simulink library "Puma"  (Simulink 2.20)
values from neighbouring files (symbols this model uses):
  a = input('Inserisci il dato da graficare [1=PIDNL 2=PD 3=PID]: ')    [grp.m]    (also in grp1.m = input('Inserisci il dato da graficare [1..3]'))
undefined symbols (not defined in the file or in its folder): b

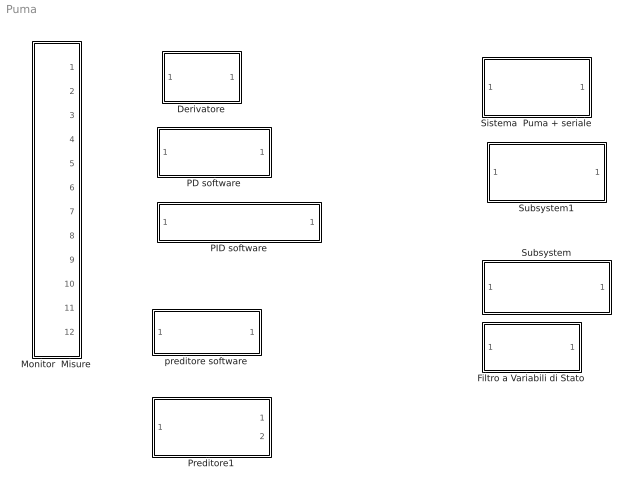
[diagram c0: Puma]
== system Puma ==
  Derivatore : Subsystem  Orientation=left  mask(Simulazione Derivatore implementato in maniera software){Td=0.13, T=0.033, N=10}
      mask prompts: Td "Costante di derivazione Td"; T "Sample Time T del PD"; N "Indice polo del derivatore [5..10]"
      mask init:
      | Kbeta=Td/(N*T+Td)
      | Kalfa=N*Kbeta
  Filtro a Variabili di Stato : Subsystem  mask{T=0.030, k1=5, k2=10}
      mask prompts: T "Sample Time"; k1 "Gudagno k1"; k2 "Guadagno k2"
      mask init:
      | A=[0,-1,-1;k1*T,1,0;0,k2*T,1];
  Monitor  Misure : Subsystem
  PD software : Subsystem  mask(Simulazione PD implementato in maniera software){Kp=0.5, Td=0.13, T=0.075, N=10}
      mask prompts: Kp "Costante guadagno proporzionale"; Td "Costante di derivazione Td"; T "Sample Time T del PD"; N "Indice polo del derivatore [5..10]"
      mask init:
      | Kbeta=Td/(N*T+Td);
      | Kalfa=N*Kbeta;
      | 
      | U0=Kbeta;
      | E1=Kp*(1+Kalfa);
      | E0=-Kp*(Kbeta+Kalfa);
  PID software : Subsystem  mask(PID simulazione di una implementazione software.){Ti=8, Td=0.17, T=.07, Kp=0.4, N=10}
      mask prompts: Ti "Costante integrativa Ti"; Td "Costante derivativa Td"; T "Sample Time del PID"; Kp "Costante proporzionale Kp"; N "Indice polo del derivatore [5..10]"
      mask init:
      | Kalfa=T/Ti;
      | Kgamma=Td/(N*T+Td);		Kbeta=N*Kgamma;
      | 
      | q0=Kp*(1+Kbeta);
      | q1=-Kp*(1+Kgamma-Kalfa+2*Kbeta);
      | q2=Kp*(Kgamma-Kalfa*Kgamma+Kbeta);
      | 
      | r1=Kgamma+1;
      | r2=Kgamma;
  Preditore1 : Subsystem  mask(Modello del Puma 260 in Alter Mode){Ts=.260}
      mask prompts: Ts "Tempo di Campionamento Ts della seriale"
      mask help: Questo blocco racchiude il comportamento dinamico del Puma 260 pilotato dalla seriale. La rappresentazione e' a variabili di stato.
      mask init:
      | K=10; % attenuazione del guadagno puma.
      | A=[0,0,0,0,0,0,0,0,0,0;
      | 1,0,0,0,0,0,0,0,0,0;
      | 0,1,0,0,0,0,0,0,0,0;
      | 0,0,1,0,0,0,0,0,0,0;
      | 0,0,0,1,0,0,0,0,0,0;
      | 0,0,0,0,1,0,0,0,0,0;
      | 0,0,0,0,0,1,0,0,0,0;
      | 0,0,0,0,0,0,1,0,0,0;
      | 0,0,0,0,0,0,0,1,0,0;
      | 0,0,0,0,0,0,0,0,1/K,1];
      | B=[1;0;0;0;0;0;0;0;0;0];
      | C=[0,0,0,0,0,0,0,0,0,1;
      | 1/K,1/K,1/K,1/K,1/K,1/K,1/K,1/K,1/K,1];
      | D=[0;0];
  Sistema  Puma + seriale : Subsystem  mask(Tempo di controllo in ms del Puma 260.){Ts=.260}
      mask prompts: Ts "Tempo di controllo del Puma [valore tipico .260 sec]"
      mask help: Blocco rappresentate il sistema formato dalla seriale (ritardo) e dal Puma 260.
  Subsystem : Subsystem  mask(Filtro di Butterworth){ordine=3, freq=0.2/16}
      mask prompts: ordine "Ordine del filtro"; freq "Parametro K per ricavare la Freq. di taglio Ft"
      mask help: Attenzione! Considerare il parametro Fc come la frequanza di campionamento del segnale di ingresso, per cui la frequanza di taglio diviene Ft=K*Fc;
      mask init:
      | [b,a]=butter(ordine,freq);
  Subsystem1 : Subsystem  mask(Modello del Puma 260 in Alter Mode){Ts=.260}
      mask prompts: Ts "Tempo di Campionamento Ts della seriale"
      mask help: Questo blocco racchiude il comportamento dinamico del Puma 260 pilotato dalla seriale. La rappresentazione e' a variabili di stato.
      mask init:
      | K=10; % attenuazione del guadagno puma.
      | A=[0,0,0,0,0,0,0,0,0,0;
      | 1,0,0,0,0,0,0,0,0,0;
      | 0,1,0,0,0,0,0,0,0,0;
      | 0,0,1,0,0,0,0,0,0,0;
      | 0,0,0,1,0,0,0,0,0,0;
      | 0,0,0,0,1,0,0,0,0,0;
      | 0,0,0,0,0,1,0,0,0,0;
      | 0,0,0,0,0,0,1,0,0,0;
      | 0,0,0,0,0,0,0,1,0,0;
      | 0,0,0,0,0,0,0,0,1/K,1];
      | B=[1;0;0;0;0;0;0;0;0;0];
      | C=[0,0,0,0,0,0,0,0,0,1];
      | D=[0];
  preditore software : Subsystem  mask(Modello dinamico preditivo del Puma 260 + ritardo seriale){Tsp=.260, Tt=.180, Tmove=.320}
      mask prompts: Tsp "Sample Time Tsp del preditore"; Tt "Ritardo Totale Tt del sistema da modellare"; Tmove "Tempo Tmove dello spostamento imposto"
      mask help: Preditore della posizione del Puma all'istante successivo. Questo viene effettuato tramite la conoscenza 1) dell'ingresso all'istante precedente 2) della posizione presente del Puma (ottenuta dalla ripresa dalla telecamera).
      mask init:
      | if exist('Tt')== 0
      | Tt=.240;
      | end
      | if exist('Tmove')== 0
      | Tmove=.320;
      | end
      | if exist('Tsp')== 0
      | Tsp=.260;
      | end

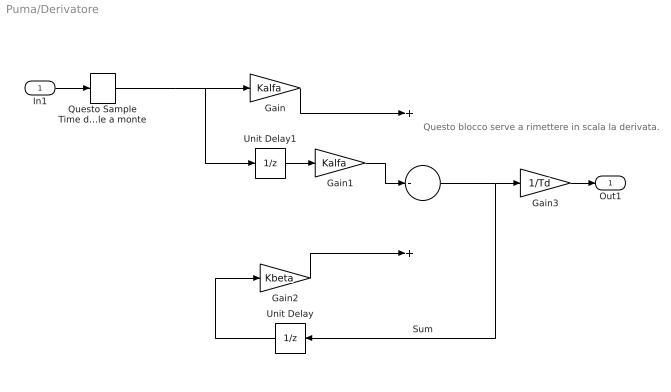
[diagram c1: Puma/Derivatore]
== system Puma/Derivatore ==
  note: Questo blocco serve a rimettere in scala la derivata.
  In1 : Inport  Port=1  PortWidth=-1  SampleTime=-1
  Gain : Gain  Gain=Kalfa
  Gain1 : Gain  Gain=Kalfa
  Gain2 : Gain  Gain=Kbeta
  Gain3 : Gain  Gain=1/Td
  Questo Sample Time deve coincidere con quello del segnale a monte : ZeroOrderHold  SampleTime=T
  Sum : Sum  Inputs=+-+
  Unit Delay : UnitDelay  Orientation=left  X0=0  SampleTime=T
  Unit Delay1 : UnitDelay  X0=0  SampleTime=T
  Out1 : Outport  Port=1
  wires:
  In1/1 -> Questo Sample Time deve coincidere con quello del segnale a monte/1
  Questo Sample Time deve coincidere con quello del segnale a monte/1 -> Gain/1, Unit Delay1/1
  Gain1/1 -> Sum/2
  Unit Delay/1 -> Gain2/1
  Gain2/1 -> Sum/3
  Gain/1 -> Sum/1
  Unit Delay1/1 -> Gain1/1
  Sum/1 -> Unit Delay/1, Gain3/1
  Gain3/1 -> Out1/1

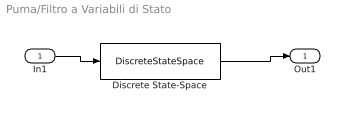
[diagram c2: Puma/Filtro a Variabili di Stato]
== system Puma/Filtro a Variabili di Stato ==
  In1 : Inport  Port=1  PortWidth=-1  SampleTime=-1
  Discrete State-Space : DiscreteStateSpace  A=A  B=[1;0;0]  C=[1,0,0;0,1,0;0,0,1]  D=[0;0;0]  X0=0  SampleTime=0.01
  Out1 : Outport  Port=1
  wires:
  In1/1 -> Discrete State-Space/1
  Discrete State-Space/1 -> Out1/1

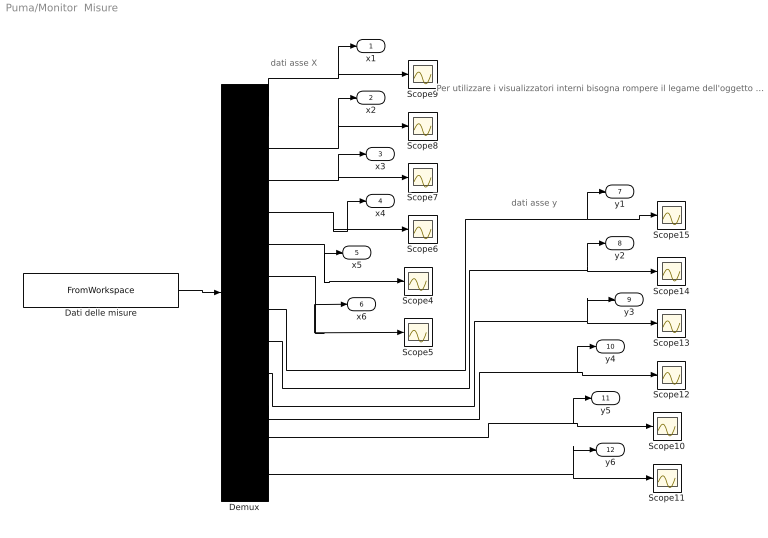
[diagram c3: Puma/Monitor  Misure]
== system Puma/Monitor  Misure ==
  note: dati asse y
  note: dati asse X
  note: Per utilizzare i visualizzatori interni bisogna rompere il legame dell'oggetto con la libreria, altrimenti utilizzare altri visualizzatori prendendo i segnali esterni Out n....
  Dati delle misure : FromWorkspace  VariableName=out
  Demux : Demux  Outputs=12
  Scope{4..15} (12 alike) : Scope
  x1 : Outport  Port=1
  x2 : Outport  Port=2
  x3 : Outport  Port=3
  x4 : Outport  Port=4
  x5 : Outport  Port=5
  x6 : Outport  Port=6
  y1 : Outport  Port=7
  y2 : Outport  Port=8
  y3 : Outport  Port=9
  y4 : Outport  Port=10
  y5 : Outport  Port=11
  y6 : Outport  Port=12
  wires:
  Dati delle misure/1 -> Demux/1
  Demux/1 -> Scope9/1, x1/1
  Demux/2 -> Scope8/1, x2/1
  Demux/3 -> Scope7/1, x3/1
  Demux/4 -> Scope6/1, x4/1
  Demux/5 -> Scope4/1, x5/1
  Demux/6 -> Scope5/1, x6/1
  Demux/12 -> Scope11/1, y6/1
  Demux/11 -> Scope10/1, y5/1
  Demux/10 -> Scope12/1, y4/1
  Demux/9 -> Scope13/1, y3/1
  Demux/8 -> Scope14/1, y2/1
  Demux/7 -> Scope15/1, y1/1

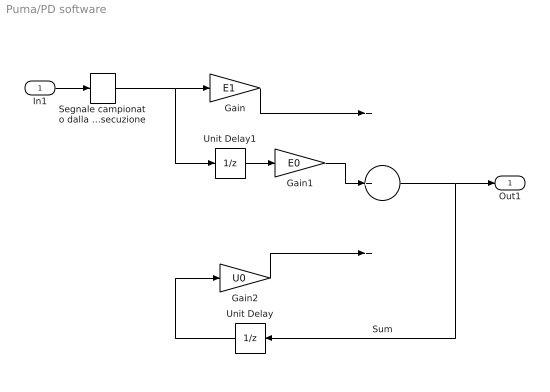
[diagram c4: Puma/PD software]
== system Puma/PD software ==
  In1 : Inport  Port=1  PortWidth=-1  SampleTime=-1
  Gain : Gain  Gain=E1
  Gain1 : Gain  Gain=E0
  Gain2 : Gain  Gain=U0
  Segnale campionato dalla procedura software al momento ciclo  di'esecuzione : ZeroOrderHold  SampleTime=T
  Sum : Sum  Inputs=+++
  Unit Delay : UnitDelay  Orientation=left  X0=0  SampleTime=T
  Unit Delay1 : UnitDelay  X0=0  SampleTime=T
  Out1 : Outport  Port=1
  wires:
  Gain1/1 -> Sum/2
  Unit Delay/1 -> Gain2/1
  Gain2/1 -> Sum/3
  Gain/1 -> Sum/1
  Unit Delay1/1 -> Gain1/1
  Sum/1 -> Out1/1, Unit Delay/1
  In1/1 -> Segnale campionato dalla procedura software al momento ciclo  di'esecuzione/1
  Segnale campionato dalla procedura software al momento ciclo  di'esecuzione/1 -> Gain/1, Unit Delay1/1

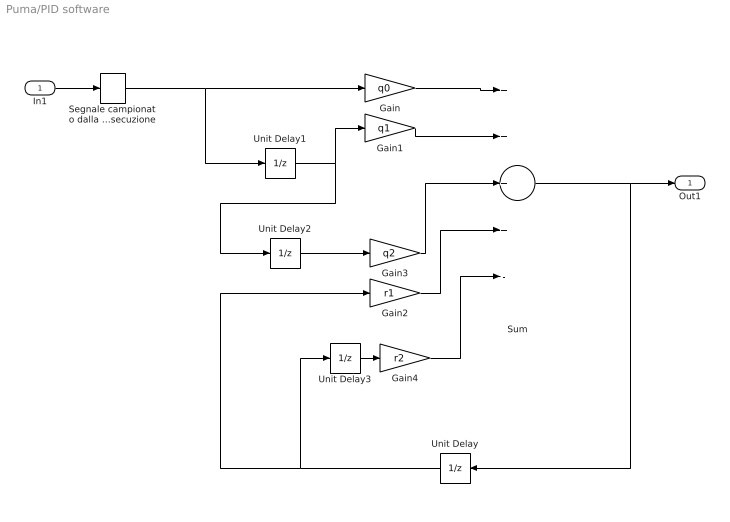
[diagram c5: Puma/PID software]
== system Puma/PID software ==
  In1 : Inport  Port=1  PortWidth=-1  SampleTime=-1
  Gain : Gain  Gain=q0
  Gain1 : Gain  Gain=q1
  Gain2 : Gain  Gain=r1
  Gain3 : Gain  Gain=q2
  Gain4 : Gain  Gain=r2
  Segnale campionato dalla procedura software al momento del  ciclo di esecuzione : ZeroOrderHold  SampleTime=T
  Sum : Sum  Inputs=++++-
  Unit Delay : UnitDelay  Orientation=left  X0=0  SampleTime=T
  Unit Delay1 : UnitDelay  X0=0  SampleTime=T
  Unit Delay2 : UnitDelay  X0=0  SampleTime=T
  Unit Delay3 : UnitDelay  X0=0  SampleTime=T
  Out1 : Outport  Port=1
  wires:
  In1/1 -> Segnale campionato dalla procedura software al momento del  ciclo di esecuzione/1
  Gain1/1 -> Sum/2
  Gain/1 -> Sum/1
  Sum/1 -> Unit Delay/1, Out1/1
  Unit Delay1/1 -> Gain1/1, Unit Delay2/1
  Unit Delay2/1 -> Gain3/1
  Gain3/1 -> Sum/3
  Gain2/1 -> Sum/4
  Unit Delay/1 -> Gain2/1, Unit Delay3/1
  Unit Delay3/1 -> Gain4/1
  Gain4/1 -> Sum/5
  Segnale campionato dalla procedura software al momento del  ciclo di esecuzione/1 -> Gain/1, Unit Delay1/1

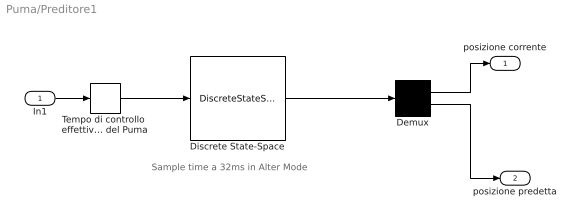
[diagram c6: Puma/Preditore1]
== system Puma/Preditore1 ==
  note: Sample time a 32ms in Alter Mode
  In1 : Inport  Port=1  PortWidth=-1  SampleTime=-1
  Demux : Demux  Outputs=2
  Discrete State-Space : DiscreteStateSpace  A=A  B=B  C=C  D=D  X0=0  SampleTime=.033
  Tempo di controllo  effettivo Ts del Puma : ZeroOrderHold  SampleTime=Ts
  posizione corrente : Outport  Port=1
  posizione predetta : Outport  Port=2
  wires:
  In1/1 -> Tempo di controllo  effettivo Ts del Puma/1
  Discrete State-Space/1 -> Demux/1
  Tempo di controllo  effettivo Ts del Puma/1 -> Discrete State-Space/1
  Demux/1 -> posizione corrente/1
  Demux/2 -> posizione predetta/1

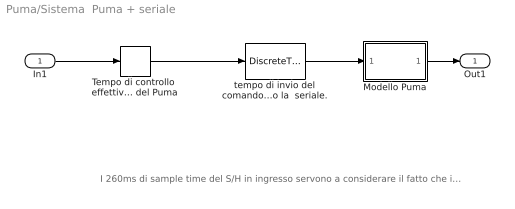
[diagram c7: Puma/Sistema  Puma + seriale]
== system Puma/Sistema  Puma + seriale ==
  note: I 260ms di sample time del S/H in ingresso servono a considerare il fatto che il controller Unival restituisce il prompt rispedendolo indietro. Quindi l'effettiva banda di controllo e' di 260ms, ma il tempo che inpiega il robot ad eseguire il comando e' di circa 8*32ms+80ms~350 ms
  In1 : Inport  Port=1  PortWidth=-1  SampleTime=-1
  Modello Puma : Subsystem  Description=Modello Puma
  Tempo di controllo  effettivo Ts del Puma : ZeroOrderHold  SampleTime=Ts
  tempo di invio del comando attraverso la  seriale. : DiscreteTransferFcn  Numerator=1  Denominator=[1 0 0 0 0 0 0 0 0]  SampleTime=.032
  Out1 : Outport  Port=1
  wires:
  tempo di invio del comando attraverso la  seriale./1 -> Modello Puma/1(In1)
  Modello Puma/1(Out1) -> Out1/1
  In1/1 -> Tempo di controllo  effettivo Ts del Puma/1
  Tempo di controllo  effettivo Ts del Puma/1 -> tempo di invio del comando attraverso la  seriale./1

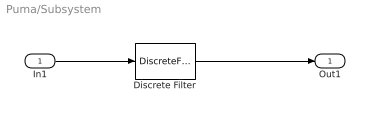
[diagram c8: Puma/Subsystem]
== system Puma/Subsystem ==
  In1 : Inport  Port=1  PortWidth=-1  SampleTime=-1
  Discrete Filter : DiscreteFilter  Numerator=b  Denominator=a  SampleTime=.032
  Out1 : Outport  Port=1
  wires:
  In1/1 -> Discrete Filter/1
  Discrete Filter/1 -> Out1/1

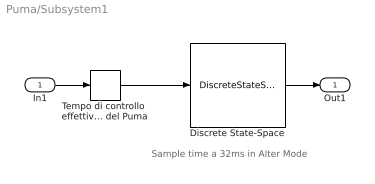
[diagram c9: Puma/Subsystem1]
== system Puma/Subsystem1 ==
  note: Sample time a 32ms in Alter Mode
  In1 : Inport  Port=1  PortWidth=-1  SampleTime=-1
  Discrete State-Space : DiscreteStateSpace  A=A  B=B  C=C  D=D  X0=0  SampleTime=.032
  Tempo di controllo  effettivo Ts del Puma : ZeroOrderHold  SampleTime=Ts
  Out1 : Outport  Port=1
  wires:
  In1/1 -> Tempo di controllo  effettivo Ts del Puma/1
  Discrete State-Space/1 -> Out1/1
  Tempo di controllo  effettivo Ts del Puma/1 -> Discrete State-Space/1

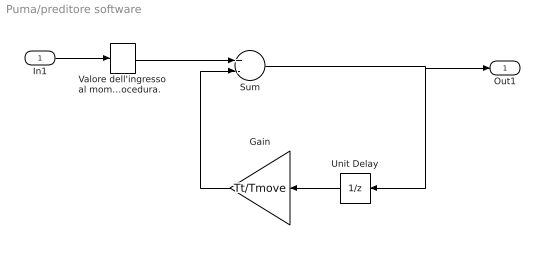
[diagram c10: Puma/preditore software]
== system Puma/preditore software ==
  In1 : Inport  Port=1  PortWidth=-1  SampleTime=-1
  Gain : Gain  Orientation=left  Gain=Tt/Tmove
  Sum : Sum  Inputs=+-
  Unit Delay : UnitDelay  Orientation=left  X0=0  SampleTime=Tsp
  "Valore dell'ingresso al momento dell'entrata  nella procedura.  " : ZeroOrderHold  SampleTime=Tsp
  Out1 : Outport  Port=1
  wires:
  Gain/1 -> Sum/2
  Unit Delay/1 -> Gain/1
  Sum/1 -> Out1/1, Unit Delay/1
  In1/1 -> "Valore dell'ingresso al momento dell'entrata  nella procedura.  "/1
  "Valore dell'ingresso al momento dell'entrata  nella procedura.  "/1 -> Sum/1

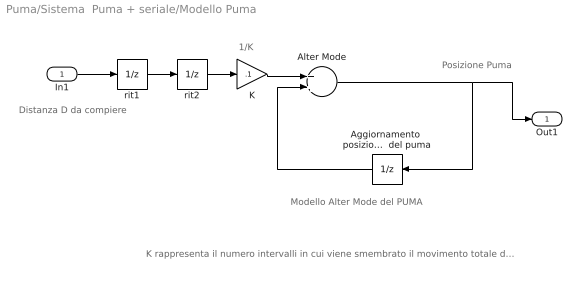
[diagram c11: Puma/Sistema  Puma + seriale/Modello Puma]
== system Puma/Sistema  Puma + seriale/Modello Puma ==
  note: Posizione Puma
  note: Modello Alter Mode del PUMA
  note: 1/K
  note: K rappresenta il numero intervalli in cui viene smembrato il movimento totale da compiere, dopo K time-slice (del PUMA) si ottiene che si e' compiuto proprio la distanza D trasmessa.
  note: Distanza D da compiere
  In1 : Inport  Port=1  PortWidth=-1  SampleTime=-1
  Aggiornamento  posizione   Il sample-time di questo blocco rappresenta la TIME-SLICE  del puma : UnitDelay  Orientation=left  X0=0  SampleTime=.032
  Alter Mode : Sum  Inputs=++
  K : Gain  Gain=.1
  rit1 : UnitDelay  X0=0  SampleTime=.032
  rit2 : UnitDelay  X0=0  SampleTime=.032
  Out1 : Outport  Port=1
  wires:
  K/1 -> Alter Mode/1
  Aggiornamento  posizione   Il sample-time di questo blocco rappresenta la TIME-SLICE  del puma/1 -> Alter Mode/2
  Alter Mode/1 -> Out1/1, Aggiornamento  posizione   Il sample-time di questo blocco rappresenta la TIME-SLICE  del puma/1
  In1/1 -> rit1/1
  rit1/1 -> rit2/1
  rit2/1 -> K/1
